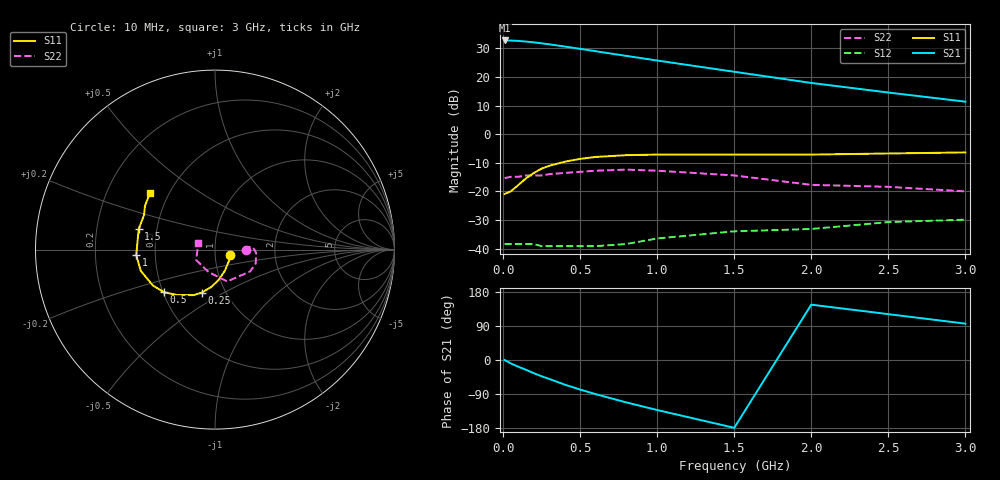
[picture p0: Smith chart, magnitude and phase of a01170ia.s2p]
!  INA-01170  S PARAMETERS
!  Id = 35 mA  LAST UPDATED 07-22-92
# ghz s ma r 50
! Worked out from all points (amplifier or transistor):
!   16 points, 10 MHz to 3 GHz, reference 50 ohm
!   highest |S21| = 32.8 dB at 10 MHz (marker M1)
!   |S21| within 3 dB of that: start of sweep to 507.7 MHz
!   unconditionally stable (mu >= 1): start of sweep to end of sweep
!   at 100 MHz: K = 1.17, MAG = 33.1 dB, |S12| = -38.4 dB
!   at 500 MHz: K = 1.35, MAG = 31.0 dB, |S12| = -39.2 dB
!   at 3 GHz: K = 3.31, MAG = 12.5 dB, |S12| = -29.9 dB
!   lowest NFmin = 1.20 dB at 100 MHz
!   S11 on the Smith chart (normalised r, x): 10 MHz: 1.18, -0.07; 250 MHz: 0.78, -0.40; 500 MHz: 0.51, -0.28; 1 GHz: 0.39, -0.03; 1.5 GHz: 0.39, +0.11; 3 GHz: 0.39, +0.32
0.01  0.09 -20.0  43.65 0.0  0.012 -5.0  0.17 -1.0
0.05  0.1 -39.0  43.51 -9.0  0.012 17.0  0.18 0.0
0.1  0.13 -65.0  42.82 -18.0  0.012 -4.0  0.18 1.0
0.15  0.17 -83.0  41.71 -26.0  0.012 17.0  0.19 2.0
0.2  0.21 -96.0  40.41 -35.0  0.012 12.0  0.19 3.0
0.25  0.25 -107.0  38.93 -43.0  0.011 26.0  0.19 4.0
0.3  0.28 -115.0  37.38 -50.0  0.011 3.0  0.2 5.0
0.4  0.33 -130.0  34.19 -65.0  0.011 21.0  0.21 3.0
0.5  0.37 -140.0  31.13 -78.0  0.011 11.0  0.22 0.0
0.6  0.4 -150.0  28.3 -90.0  0.011 22.0  0.23 -5.0
0.8  0.43 -164.0  23.43 -112.0  0.012 30.0  0.24 -19.0
1  0.44 -176.0  19.45 -132.0  0.015 32.0  0.23 -32.0
1.5  0.44 165.0  12.37 -179.0  0.02 42.0  0.19 -69.0
2  0.44 154.0  7.88 146.0  0.022 42.0  0.13 -106.0
2.5  0.46 148.0  5.36 121.0  0.029 36.0  0.12 -151.0
3  0.48 139.0  3.71 96.0  0.032 45.0  0.1 159.0
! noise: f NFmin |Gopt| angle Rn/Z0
0.1  1.2  0.15  5  0.19
0.5  1.3  0.11  29  0.19
1  1.6  0.06  99  0.19
2  2.6  0.24  -158  0.2
